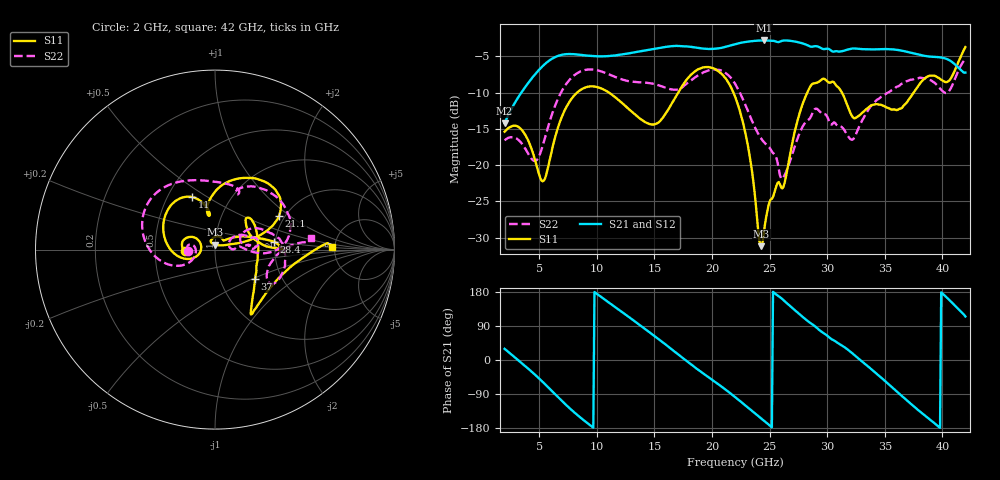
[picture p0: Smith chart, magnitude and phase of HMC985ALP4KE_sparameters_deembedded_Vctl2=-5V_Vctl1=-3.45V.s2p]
!s2p File: Measurements: S11, S21, S12, S22
# GHz S dB R 50.0
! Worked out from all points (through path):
!   401 points, 2 GHz to 42 GHz, reference 50 ohm
!   highest |S21| = -2.82 dB at 24.5 GHz (marker M1); lowest = -14.2 dB at 2 GHz (marker M2)
!   lowest |S11| = -31.2 dB at 24.3 GHz (marker M3), VSWR 1.06, Z = 50.1 + j2.77 ohm
!   |S11| at or under -10 dB: start of sweep to 8.288 GHz; 21.86 GHz to 28.27 GHz (6.412 GHz wide, 25.6 % of centre); 31.28 GHz to 37.5 GHz (6.217 GHz wide, 18.1 % of centre)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
!   |S22| runs from -21.9 to -5.3 dB; largest |S21 - S12| = 0.00063
!   S11 on the Smith chart (normalised r, x): 2 GHz: 0.71, -0.02; 11 GHz: 0.66, +0.43; 21.1 GHz: 1.86, +0.84; 28.4 GHz: 1.97, +0.19; 37 GHz: 1.47, -0.52; 42 GHz: 4.70, +0.28
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2  -15.39 -176.5  -14.23 29.5  -14.24 29.5  -16.57 -176.0
3.5  -15.16 158.7  -9.89 -8.7  -9.89 -8.7  -17.04 168.1
5.4  -22.14 -179.7  -6.21 -60.6  -6.21 -60.6  -16.81 -155.0
6.9  -13.60 -169.8  -4.82 -105.8  -4.82 -105.8  -9.97 -169.9
8.7  -9.53 146.8  -4.83 -154.9  -4.83 -154.9  -7.02 153.2
11  -9.94 113.3  -4.97 152.7  -4.98 152.7  -7.46 116.3
13.4  -13.11 99.4  -4.42 99.8  -4.42 99.8  -8.54 83.5
15.4  -14.07 101.7  -3.87 54.3  -3.87 54.3  -9.02 67.7
17.9  -8.03 76.5  -3.66 -4.9  -3.66 -4.8  -8.67 67.8
21.1  -7.89 27.8  -3.73 -76.2  -3.73 -76.2  -7.21 15.6
22  -10.51 19.5  -3.34 -97.7  -3.34 -97.6  -8.78 1.8
23.1  -17.16 15.2  -2.99 -124.9  -2.99 -124.9  -12.44 -4.3
24.3  -31.15 87.0  -2.83 -154.9  -2.83 -154.8  -16.40 4.6
24.5  -29.37 108.8  -2.82 -159.9  -2.82 -159.9  -16.80 6.0
26.2  -23.00 45.5  -2.83 158.2  -2.83 158.3  -21.67 21.3
28.4  -9.57 7.5  -3.56 100.8  -3.56 100.8  -13.71 18.9
28.7  -8.81 2.5  -3.68 94.7  -3.68 94.7  -12.89 17.5
32.4  -13.54 27.6  -3.93 12.0  -3.93 12.0  -16.07 26.1
35.4  -12.19 14.5  -4.02 -65.6  -4.02 -65.5  -9.91 17.0
37  -11.16 -36.0  -4.41 -108.7  -4.41 -108.6  -8.39 3.8
39.7  -7.99 -55.4  -5.13 -176.5  -5.13 -176.4  -9.28 -31.2
42  -3.74 1.5  -7.25 114.8  -7.25 114.8  -5.33 6.7
